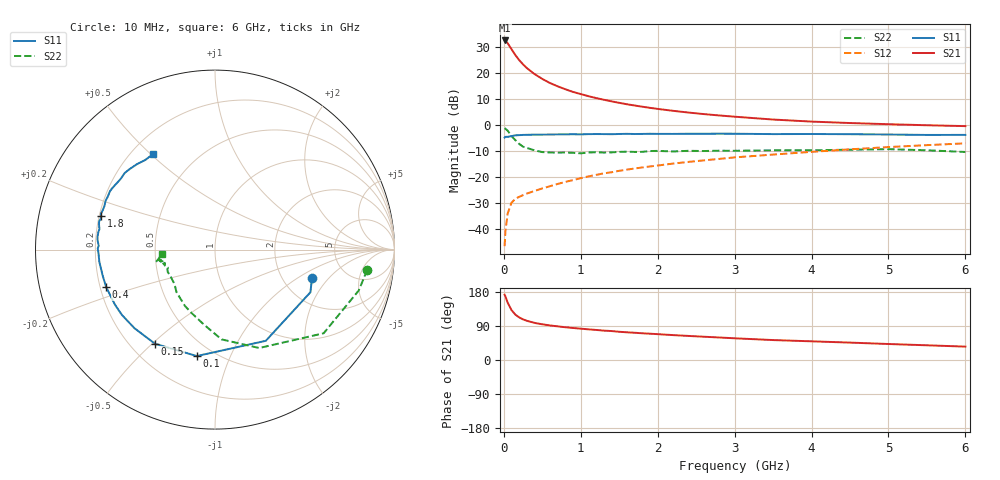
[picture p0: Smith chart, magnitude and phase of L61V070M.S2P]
!  INFINEON TECHNOLOGIES Small Signal Semiconductors
! BFR380L3 , Si-NPN RF-Transistor in TSLP-3-1
!  Vce=1 V,  Ic=70 mA
! Common Emitter S-Parameters:  07. March 2005
#  GHz  S  MA  R  50
! f  S11  S21  S12  S22
! GHz  Mag  Ang  Mag  Ang  Mag  Ang  Mag  Ang
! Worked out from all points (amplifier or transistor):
!   36 points, 10 MHz to 6 GHz, reference 50 ohm
!   highest |S21| = 32.4 dB at 10 MHz (marker M1)
!   |S21| within 3 dB of that: start of sweep to 91.78 MHz
!   unconditionally stable (mu >= 1): 885.5 MHz to end of sweep
!   at 250 MHz: K = 0.56, MSG = 25.1 dB, |S12| = -27.1 dB
!   at 1.4 GHz: K = 1.07, MAG = 12.0 dB, |S12| = -18.3 dB
!   at 6 GHz: K = 1.01, MAG = 2.6 dB, |S12| = -7.2 dB
!   S11 on the Smith chart (normalised r, x): 10 MHz: 2.90, -1.33; 100 MHz: 0.41, -0.76; 150 MHz: 0.30, -0.51; 400 MHz: 0.22, -0.16; 1.8 GHz: 0.21, +0.14; 6 GHz: 0.29, +0.51
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0.01  0.563 -16.1  41.48 172.2  0.0046 71.4  0.8555 -7.6
0.02  0.5823 -24.1  41.02 168.0  0.0087 75.0  0.8326 -15.9
0.05  0.5817 -60.9  36.66 151.1  0.0196 64.3  0.764 -37.6
0.1  0.6017 -99.7  28.11 131.6  0.0315 52.4  0.6011 -65.8
0.15  0.622 -122.5  21.69 119.6  0.0376 46.9  0.5016 -85.8
0.2  0.6271 -135.7  17.34 112.4  0.0409 45.6  0.4249 -97.9
0.25  0.6337 -145.0  14.38 107.2  0.0441 44.4  0.3763 -110.4
0.3  0.6363 -151.4  12.18 103.4  0.0473 46.3  0.3558 -118.1
0.4  0.6413 -160.9  9.343 97.9  0.0531 48.7  0.3195 -132.2
0.5  0.6423 -166.9  7.558 94.2  0.0593 51.8  0.2963 -139.6
0.6  0.6445 -171.0  6.297 91.2  0.0654 53.9  0.2911 -145.2
0.7  0.6481 -174.1  5.441 88.8  0.0723 56.4  0.2888 -150.6
0.9  0.6533 179.4  4.249 84.5  0.0858 59.5  0.2864 -157.9
1.1  0.656 175.6  3.519 80.9  0.1011 61.6  0.2909 -160.2
1.4  0.6535 170.0  2.8 76.4  0.1213 63.1  0.2922 -163.9
1.8  0.6618 163.6  2.208 70.5  0.1501 63.9  0.2993 -167.6
2.2  0.6622 158.5  1.841 65.7  0.1782 63.9  0.3044 -168.1
2.8  0.6694 151.0  1.5 59.4  0.2192 63.6  0.315 -170.7
3.5  0.6568 143.1  1.251 52.6  0.2655 61.1  0.3203 -169.6
4.5  0.6537 136.6  1.072 45.9  0.3346 58.6  0.3291 -168.9
5.5  0.6328 128.0  0.972 38.8  0.4029 53.9  0.3209 -170.3
6  0.6341 122.9  0.935 35.3  0.4362 51.4  0.2976 -175.2
